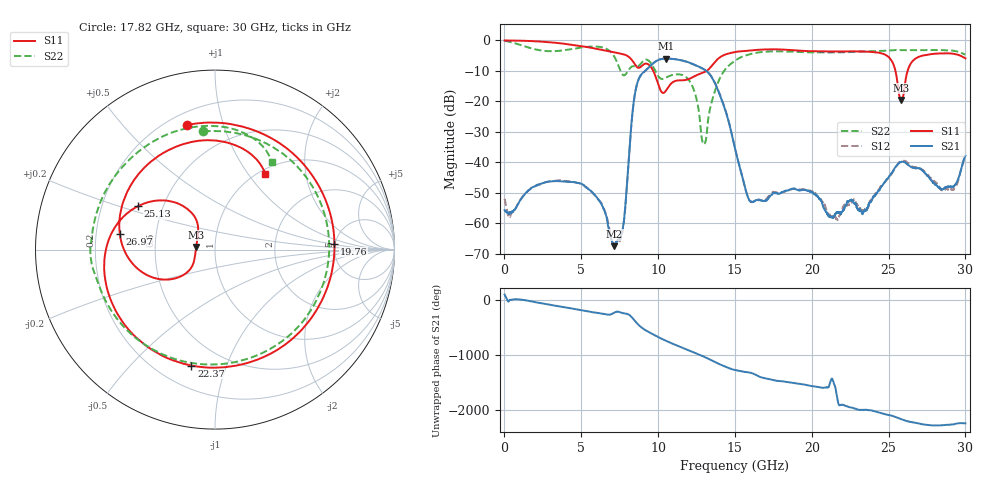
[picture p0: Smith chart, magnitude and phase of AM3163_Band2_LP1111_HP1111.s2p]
!Agilent Technologies,E8364B,MY43040894,A.07.50.67
!Agilent E8364B: A.07.50.67
!Date: Thursday, August 20, 2020 11:13:22
!Correction: S11(Full 2 Port(1,2))
!S21(Full 2 Port(1,2))
!S12(Full 2 Port(1,2))
!S22(Full 2 Port(1,2))
!S2P File: Measurements: S11, S21, S12, S22:
# Hz S  dB  R 50
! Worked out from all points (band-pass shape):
!   3201 points, 10 MHz to 30 GHz, reference 50 ohm
!   highest |S21| = -5.96 dB at 10.54 GHz (marker M1); lowest = -67.6 dB at 7.142 GHz (marker M2)
!   |S21| within 3 dB of the highest: 9.377 GHz to 12.78 GHz (3.407 GHz wide, 30.8 % of centre)
!   lowest |S11| = -19.5 dB at 25.83 GHz (marker M3), VSWR 1.24, Z = 40.5 + j1.15 ohm
!   |S11| at or under -10 dB: 9.682 GHz to 13.17 GHz (3.489 GHz wide, 30.5 % of centre); 25.45 GHz to 26.24 GHz (791 MHz wide, 3.06 % of centre)
!   |S22| runs from -34.1 to -0.1 dB; largest |S21 - S12| = 0.0071
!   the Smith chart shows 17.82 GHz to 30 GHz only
!   S11 on the Smith chart (normalised r, x): 17.82 GHz: 0.27, +0.76; 19.76 GHz: 4.92, +0.59; 22.37 GHz: 0.33, -0.76; 25.13 GHz: 0.36, +0.23; 26.97 GHz: 0.30, +0.07; 30 GHz: 1.07, +1.22
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1e7  -0.03 -2.5  -55.72 102.3  -52.00 -28.3  -0.12 -6.6
9.190719e8  -0.10 -32.4  -53.46 14.0  -53.54 13.5  -1.31 -84.1
1.996838e9  -0.30 -70.3  -47.85 -36.1  -47.80 -34.8  -2.93 -171.4
3.421362e9  -0.85 -120.8  -46.18 -106.5  -46.05 -107.7  -3.49 85.5
5.014581e9  -1.90 179.7  -47.11 175.6  -47.25 173.6  -2.35 -16.3
7.141997e9  -3.92 75.7  -67.55 131.8  -67.34 -1.5  -5.28 -177.7
7.732425e9  -4.54 34.1  -60.57 122.1  -61.17 127.5  -11.41 57.3
8.604009e9  -8.66 -32.2  -14.77 -54.3  -14.87 -54.0  -8.57 -97.6
1.000979e10  -14.46 -141.9  -6.45 47.6  -6.46 48.0  -11.77 -175.3
1.054399e10  -16.25 -132.9  -5.96 -24.6  -5.98 -24.1  -12.13 -169.6
1.17717e10  -13.03 99.6  -6.87 -169.1  -6.89 -168.7  -11.89 135.7
1.299005e10  -10.50 -22.5  -9.51 49.5  -9.52 50.6  -34.12 -85.3
1.5005e10  -3.84 -125.4  -35.48 167.6  -35.42 166.9  -6.67 -111.8
1.781656e10  -2.96 102.6  -50.37 -31.3  -50.10 -32.3  -3.59 95.6
1.975654e10  -3.52 2.9  -49.44 -111.2  -49.24 -109.7  -3.92 2.2
2.000958e10  -3.57 -9.1  -49.73 -126.3  -49.52 -121.9  -3.96 -8.9
2.237129e10  -3.62 -101.5  -52.82 -141.8  -54.03 -137.4  -3.85 -94.6
2.500479e10  -5.48 158.1  -44.87 67.3  -44.91 68.3  -3.36 -166.4
2.512662e10  -6.15 150.6  -44.06 60.6  -44.30 59.0  -3.29 -169.4
2.582952e10  -19.53 172.4  -39.82 -8.5  -39.69 -6.0  -3.22 171.5
2.697288e10  -5.39 170.7  -41.91 -86.6  -41.86 -86.9  -3.20 142.3
3e10  -5.89 56.4  -37.88 -84.4  -37.99 -83.4  -4.70 56.9
